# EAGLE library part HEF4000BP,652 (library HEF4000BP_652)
NOR GATE Source: Datasheet
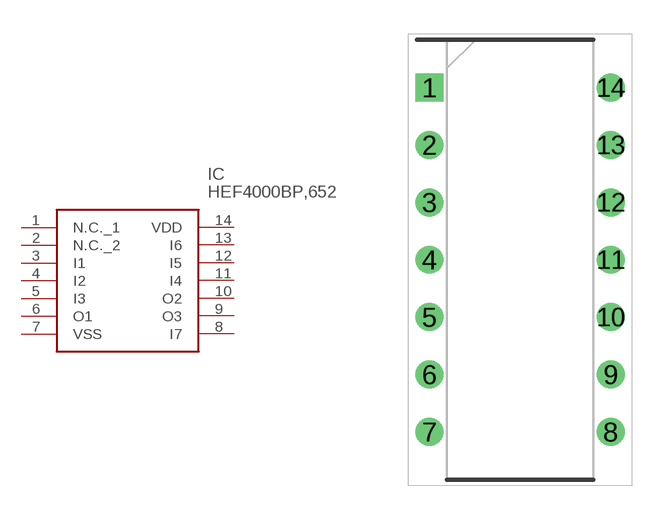
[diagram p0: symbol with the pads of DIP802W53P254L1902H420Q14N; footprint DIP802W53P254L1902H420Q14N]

Designator prefix IC

## HEF4000BP,652 (Description: NOR GATE; Height: 4.2mm; Manufacturer_Name: NXP; Manufacturer_Part_Number: HEF4000BP,652)  [DIP802W53P254L1902H420Q14N]
1  N.C._1
2  N.C._2
3  I1
4  I2
5  I3
6  O1
7  VSS
8  I7
9  O3
10  O2
11  I4
12  I5
13  I6
14  VDD

## Footprint DIP802W53P254L1902H420Q14N (pad centres in mm)
SOT27-1
drill 0.73 pad 1.13 square: 1 -4.012,7.62
drill 0.73 pad 1.13: 2 -4.012,5.08; 3 -4.012,2.54; 4 -4.012,0; 5 -4.012,-2.54; 6 -4.012,-5.08; 7 -4.012,-7.62; 8 4.012,-7.62; 9 4.012,-5.08; 10 4.012,-2.54; 11 4.012,0; 12 4.012,2.54; 13 4.012,5.08; 14 4.012,7.62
